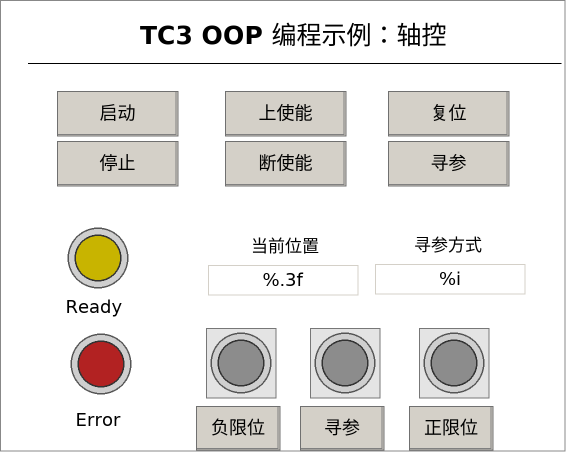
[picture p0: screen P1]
VISUALIZATION P1  // 566x452
    Button (225,91 121x45), "上使能"
        tap MAIN.bPowerOn
    Button (225,141 121x45), "断使能"
        tap MAIN.bPowerOff
    Button (57,91 121x45), "启动"
        tap MAIN.bMove
    Button (57,141 121x45), "停止"
        tap MAIN.bStop
    Button (388,91 121x45), "复位", text variable: MAIN.bReset
        tap MAIN.bReset
    Button (388,141 121x45), "寻参", text variable: MAIN.bHome
        tap MAIN.bHome
    Lamp1 (63,223 70x70), variable: MAIN.Status.Axis_Ready, style: Lamp-Lamp1-Yellow
    Lamp1 (66,329 70x70), variable: MAIN.Status.Axis_Err, style: Lamp-Lamp1-Red
    Label (23,405 150x30), "Error"
    Label (19,292 150x30), "Ready"
    PushSwitch (310,328 70x70), variable: MAIN.DrvIn.HomeSensor, behaviour: TOGGLE, style: Switch-PushSwitch-Gray
    PushSwitch (206,328 70x70), variable: MAIN.DrvIn.Limit_Neg, behaviour: TOGGLE, style: Switch-PushSwitch-Gray
    PushSwitch (419,328 70x70), variable: MAIN.DrvIn.Limit_Pos, behaviour: TOGGLE, style: Switch-PushSwitch-Gray
    Button (300,406 84x44), "寻参", text variable: MAIN.DrvIn.HomeSensor
        tap MAIN.DrvIn.HomeSensor
    Button (196,406 84x44), "负限位", text variable: MAIN.DrvIn.Limit_Neg
        tap MAIN.DrvIn.HomeSensor
    Button (409,406 84x44), "正限位", text variable: MAIN.DrvIn.Limit_Pos
        tap MAIN.DrvIn.HomeSensor
    Label (210,231 150x30), "当前位置"
    Textfield (208,265 150x30), "%.3f", text variable: MAIN.Status.Current_Pos
    Label (23,4 541x62), "TC3 OOP 编程示例：轴控"
    Line (28,63) (561,63)
    Textfield (375,264 150x30), "%i", text variable: MAIN.PARA.HomingMode
        OnMouseClick: write the text variable via Default, min 0, max 1
    Label (373,230 150x30), "寻参方式"
END_VISUALIZATION
